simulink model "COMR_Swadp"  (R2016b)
settings: Solver=FixedStepDiscrete  StartTime=0.0  StopTime=10.0  FixedStep=0.02  RelTol=1e-3  EnableMultiTasking=on
undefined symbols (not defined in the file or in its folder): bin2dec, COMR_ahBattNrmCap_C, COMR_cntNvmReadErr_CW, COMR_ti638LinComErr_C, COMR_tiNvmReadErr_C
libraries: simulink x93, dspswit3 x2
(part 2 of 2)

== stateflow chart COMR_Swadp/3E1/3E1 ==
  state Cell_Volt
    state CellVolt
      en:
      COMR_tCellTempA = BSPR_tBattTemp_A[j];
      COMR_tCellTempB = BSPR_tBattTemp_A[j+1];
      COMR_tCellTempC = BSPR_tBattTemp_A[j+2];
      COMR_tCellTempD = BSPR_tBattTemp_A[j+3];
      COMR_tCellTempE = BSPR_tBattTemp_A[j+4];
      COMR_tCellTempF = BSPR_tBattTemp_A[j+5];
      COMR_tCellTempG = BSPR_tBattTemp_A[j+6];
      BSPR_cntCellTemp = j/7;
    state CellVolt1
      en:
      j= j+7;
      COMR_tCellTempA = BSPR_tBattTemp_A[j];
      COMR_tCellTempB = 0;
      COMR_tCellTempC = 0;
      COMR_tCellTempD = 0;
      COMR_tCellTempE = 0;
      COMR_tCellTempF = 0;
      COMR_tCellTempG = 0;
      BSPR_cntCellTemp = j/7;
    state CellVolt2
      en:
      j = j+7;
      COMR_tCellTempA = BSPR_tBattTemp_A[j];
      COMR_tCellTempB = BSPR_tBattTemp_A[j+1];
      COMR_tCellTempC = 0;
      COMR_tCellTempD = 0;
      COMR_tCellTempE = 0;
      COMR_tCellTempF = 0;
      COMR_tCellTempG = 0;
      BSPR_cntCellTemp = j/7;
    state CellVolt3
      en:
      j = j+7;
      COMR_tCellTempA = BSPR_tBattTemp_A[j];
      COMR_tCellTempB = BSPR_tBattTemp_A[j+1];
      COMR_tCellTempC = BSPR_tBattTemp_A[j+2];
      COMR_tCellTempD = 0;
      COMR_tCellTempE = 0;
      COMR_tCellTempF = 0;
      COMR_tCellTempG = 0;
      BSPR_cntCellTemp = j/7;
    state CellVolt4
      en:
      j = j+7;
      COMR_tCellTempA = BSPR_tBattTemp_A[j];
      COMR_tCellTempB = BSPR_tBattTemp_A[j+1];
      COMR_tCellTempC = BSPR_tBattTemp_A[j+2];
      COMR_tCellTempD = BSPR_tBattTemp_A[j+3];
      COMR_tCellTempE = 0;
      COMR_tCellTempF = 0;
      COMR_tCellTempG = 0;
      BSPR_cntCellTemp = j/7;
    state CellVolt5
      en:
      j = j+7;
      COMR_tCellTempA = BSPR_tBattTemp_A[j];
      COMR_tCellTempB = BSPR_tBattTemp_A[j+1];
      COMR_tCellTempC = BSPR_tBattTemp_A[j+2];
      COMR_tCellTempD = BSPR_tBattTemp_A[j+3];
      COMR_tCellTempE = BSPR_tBattTemp_A[j+4];
      COMR_tCellTempF = 0;
      COMR_tCellTempG = 0;
      BSPR_cntCellTemp = j/7;
    state CellVolt6
      en:
      j = j+7;
      COMR_tCellTempA = BSPR_tBattTemp_A[j];
      COMR_tCellTempB = BSPR_tBattTemp_A[j+1];
      COMR_tCellTempC = BSPR_tBattTemp_A[j+2];
      COMR_tCellTempD = BSPR_tBattTemp_A[j+3];
      COMR_tCellTempE = BSPR_tBattTemp_A[j+4];
      COMR_tCellTempF = BSPR_tBattTemp_A[j+5];
      COMR_tCellTempG = 0;
      BSPR_cntCellTemp = j/7;
    (default) -> (junction 97)
    (junction 175) -> (junction 97)
    (junction 154) -> (junction 175)
    (junction 97) -> CellVolt : {j = 0;}
    (junction 149) -> CellVolt : {j = j + 7;}
    (junction 152) -> (junction 149)
    CellVolt -> (junction 152)
    CellVolt -> (junction 154) : [BSPR_cntBattTSnsrNum - j == 7]
    (junction 172) -> (junction 154)
    CellVolt -> CellVolt1 : [ (BSPR_cntBattTSnsrNum - j == 8)  ]
    CellVolt -> CellVolt2 : [ (BSPR_cntBattTSnsrNum - j == 9)  ]
    CellVolt -> CellVolt3 : [(BSPR_cntBattTSnsrNum - j == 10)  ]
    CellVolt -> CellVolt4 : [(BSPR_cntBattTSnsrNum - j == 11)  ]
    CellVolt -> CellVolt5 : [ (BSPR_cntBattTSnsrNum - j == 12)  ]
    CellVolt -> CellVolt6 : [(BSPR_cntBattTSnsrNum - j == 13)  ]
    CellVolt1 -> (junction 114)
    CellVolt2 -> (junction 157)
    CellVolt3 -> (junction 159)
    CellVolt4 -> (junction 161)
    CellVolt5 -> (junction 163)
    CellVolt6 -> (junction 166)
    (junction 114) -> (junction 172)
    (junction 157) -> (junction 114)
    (junction 159) -> (junction 157)
    (junction 161) -> (junction 159)
    (junction 163) -> (junction 161)
    (junction 166) -> (junction 163)
  data: BSPR_tBattTemp_A input; i local uint8; BSPR_cntCellTemp output uint8; COMR_tCellTempA output single; COMR_tCellTempB output single; COMR_tCellTempC output single; COMR_tCellTempD output single; COMR_tCellTempE output single; COMR_tCellTempF output single; j local uint8; COMR_tCellTempG output single; BSPR_cntBattTSnsrNum input

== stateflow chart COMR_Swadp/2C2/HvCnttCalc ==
  state Discnnt_Stt
    entry:
    BCCR_stHVConnSt=uint8(0);
    COMR_tiHvCnntStCalc=single(0);
  state Cnnting_Stt
    entry:
    BCCR_stHVConnSt=uint8(1);
  state DisCnntConfirm_Stt
    entry:
    BCCR_stHVConnSt=uint8(2);
    COMR_tiHvCnntStCalc=single(0);
    during:
    COMR_tiHvCnntStCalc=COMR_tiHvCnntStCalc+single(0.01);
  state Cnnt_Stt
    entry:
    BCCR_stHVConnSt=uint8(2);
  (default) -> Discnnt_Stt
  Discnnt_Stt -> Cnnting_Stt : [BCCR_stBmsCtrMode==3]
  Cnnting_Stt -> Discnnt_Stt : [BCCR_stBmsCtrMode==14||... BCCR_stBmsCtrMode==17]
  DisCnntConfirm_Stt -> Discnnt_Stt : [BCCR_stMainCtrDisConn==1||... BCCR_stMainCtrDisConn==2||... COMR_tiHvCnntStCalc>=1||... COMR_stPwrUpDwnVcuReq==1]
  Cnnting_Stt -> Cnnt_Stt : [BCCR_stBmsCtrMode==4]
  Cnnt_Stt -> DisCnntConfirm_Stt : [BCCR_stBmsCtrMode==5||... BCCR_stBmsCtrMode==7]
  data: BCCR_stBmsCtrMode input uint8; COMR_stPwrUpDwnVcuReq input uint8; BCCR_stHVConnSt output uint8; COMR_tiHvCnntStCalc local single; BCCR_stMainCtrDisConn input uint8
